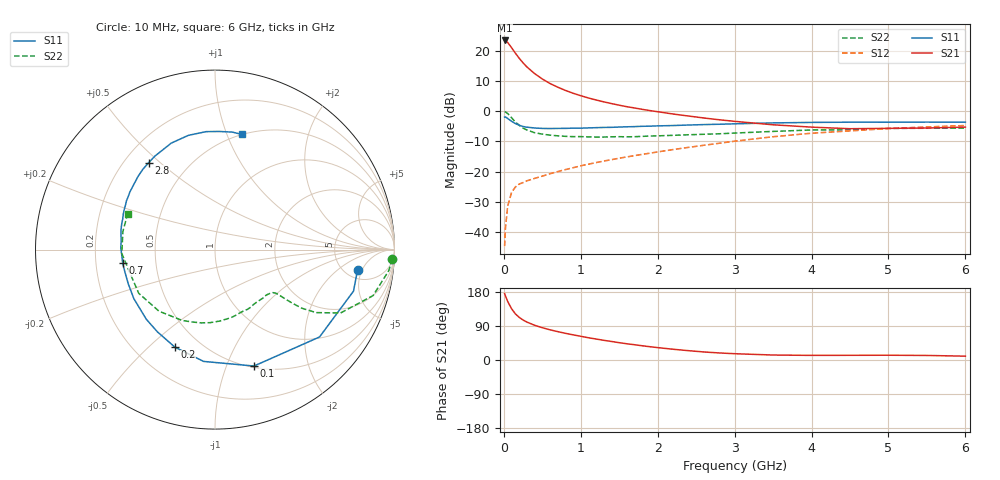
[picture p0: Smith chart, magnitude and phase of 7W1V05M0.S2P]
! Infineon Technologies  Discrete & RF Semiconductors
! BFS17W
! Si NPN RF Bipolar Junction Transistor in SOT323
! VCE = 1 V  IC = 5 mA
! Common Emitter S-Parameters:  August  1999
# GHz  S  MA  R  50
!  f  S11  S21  S12  S22
! GHz  MAG  ANG  MAG  ANG  MAG  ANG  MAG  ANG
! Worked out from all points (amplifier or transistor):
!   36 points, 10 MHz to 6 GHz, reference 50 ohm
!   highest |S21| = 23.5 dB at 10 MHz (marker M1)
!   |S21| within 3 dB of that: start of sweep to 117.1 MHz
!   unconditionally stable (mu >= 1): 491.7 MHz to end of sweep
!   at 250 MHz: K = 0.62, MSG = 19.8 dB, |S12| = -23.6 dB
!   at 1.4 GHz: K = 1.33, MAG = 5.8 dB, |S12| = -16.0 dB
!   at 6 GHz: K = 1.12, MAG = -2.4 dB, |S12| = -4.7 dB
!   S11 on the Smith chart (normalised r, x): 10 MHz: 6.42, -4.13; 100 MHz: 0.51, -1.26; 200 MHz: 0.37, -0.61; 700 MHz: 0.32, -0.07; 2.8 GHz: 0.30, +0.46; 6 GHz: 0.50, +1.13
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0.01  0.8024 -8.2  14.93 175.3  0.0058 82.2  0.9892 -3.0
0.02  0.8056 -16.7  14.89 169.4  0.0112 83.1  0.9753 -6.9
0.05  0.759 -39.9  13.8 154.5  0.0268 70.7  0.9174 -16.2
0.1  0.6841 -71.5  11.36 135.4  0.045 57.6  0.7835 -26.8
0.15  0.6262 -95.8  9.199 121.7  0.0555 49.3  0.6644 -31.9
0.2  0.5875 -112.4  7.561 112.5  0.0621 46.2  0.5845 -34.0
0.25  0.5594 -125.0  6.339 105.5  0.0658 43.8  0.5257 -34.7
0.3  0.5451 -134.6  5.43 100.1  0.0703 43.6  0.4896 -35.0
0.4  0.5283 -148.9  4.214 91.6  0.0772 44.1  0.4408 -35.3
0.5  0.5195 -158.4  3.43 85.2  0.0841 45.6  0.4177 -35.6
0.6  0.5172 -165.8  2.888 79.7  0.0921 47.6  0.402 -36.6
0.7  0.5197 -171.6  2.511 74.9  0.1 49.7  0.3919 -38.5
0.9  0.5249 179.1  1.991 66.4  0.1158 51.8  0.3796 -43.0
1.1  0.5301 171.0  1.661 58.7  0.1327 53.5  0.3761 -48.5
1.3  0.5395 164.3  1.432 51.9  0.1497 54.5  0.3738 -55.1
1.6  0.553 156.0  1.19 42.8  0.175 55.6  0.377 -65.0
2.2  0.5801 141.2  0.901 28.4  0.2318 56.3  0.3992 -86.4
2.8  0.6093 127.3  0.723 18.6  0.295 54.2  0.4237 -108.1
3.5  0.6415 112.3  0.597 13.1  0.3783 49.0  0.4639 -132.3
4.5  0.6591 94.3  0.514 12.4  0.4728 37.4  0.4924 -165.3
5.5  0.6617 81.6  0.528 12.0  0.5497 26.5  0.5229 169.0
6  0.659 76.7  0.546 10.1  0.581 21.1  0.5262 157.7
